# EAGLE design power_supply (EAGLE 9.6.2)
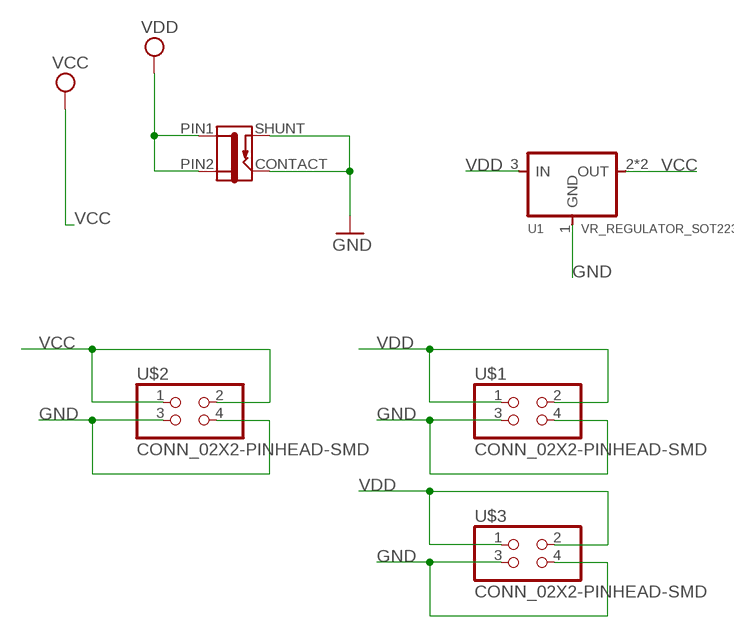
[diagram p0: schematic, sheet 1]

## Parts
J1  CONN_JACK-2.1MM  [PJ-002AH-SMT]
U1  VR_REGULATOR_SOT223  [SOT223]
U$1  CONN_02X2-PINHEAD-SMD  [2X02SMD]
U$2  CONN_02X2-PINHEAD-SMD  [2X02SMD]
U$3  CONN_02X2-PINHEAD-SMD  [2X02SMD]

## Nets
GND: J1.CONTACT J1.SHUNT U1.1(GND) U$1.3 U$1.4 U$2.3 U$2.4 U$3.3 U$3.4
VCC: U1.2(OUT) U1.4(OUT) U$2.1 U$2.2
VDD: J1.PIN1 J1.PIN2 U1.3(IN) U$1.1 U$1.2 U$3.1 U$3.2

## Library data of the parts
J1 = fab:CONN_JACK-2.1MM: SMD DC power jack PJ-002AH-SMT As found in the fablab inventory. Made by Zaerc.
U1 = fab:VR_REGULATOR_SOT223
U$1-U$3 = fab:CONN_02X2-PINHEAD-SMD

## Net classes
0 default: width 0.508 mm, clearance 0.508 mm

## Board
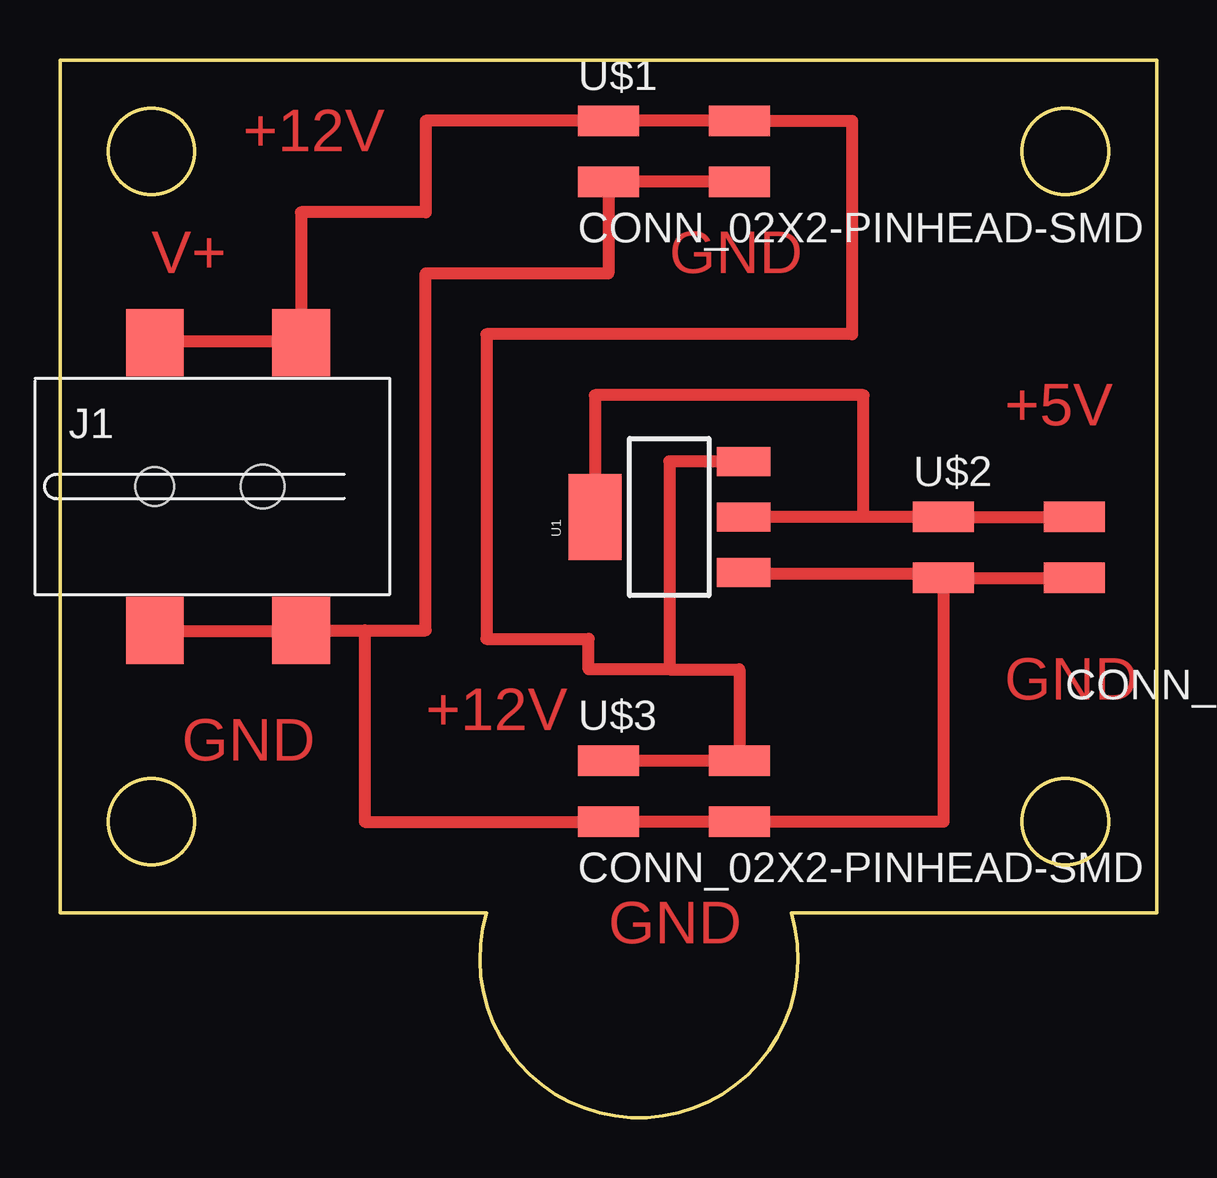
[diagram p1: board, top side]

Size 45.72 x 44.09 mm. Coordinates in mm from the lower left corner, seen from the top.
Outline: 45.72,8.53 45.72,44.09 0,44.09 0,8.53 17.78,8.53 arc213 30.48,8.53 45.72,8.53
Outline: circle at 3.81,12.34 radius 1.8
Outline: circle at 3.81,40.28 radius 1.8
Outline: circle at 41.91,40.28 radius 1.8
Outline: circle at 41.91,12.34 radius 1.8
Copper layers (1*16): Top 0.035mm / dielectric 1.5mm / Bottom 0.035mm
Design rules "default": minimum track width 6mil, minimum drill 0.35mm, track to track 6mil, track to pad 6mil, pad to pad 6mil, via to via 6mil, smd to smd 6mil, copper to edge 40mil, drill to drill 6mil, minimum pad ring 10mil, minimum via ring 8mil, stop-mask expansion 4mil, vias tented up to drill 0mil, thermal gap 10mil

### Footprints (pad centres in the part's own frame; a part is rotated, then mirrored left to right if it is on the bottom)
PJ-002AH-SMT = smd 2.4 x 2.8: CONTACT -2.4,-6; PIN1 3.7,6; PIN2 -2.4,6; SHUNT 3.7,-6 | hole 1.6: -2.4,0 | hole 1.8: 2.1,0
SOT223 = smd 1.219 x 2.235: 1 -2.311,-3.099; 2 0,-3.099; 3 2.311,-3.099 | smd 3.6 x 2.2: 4 0,3.099
2X02SMD = smd 2.54 x 1.27: 1 -2.54,1.27; 2 2.92,1.27; 3 -2.54,-1.27; 4 2.92,-1.27

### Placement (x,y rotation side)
J1  6.35,26.31 0 top
U1  25.4,25.04 90 top
U$1  25.4,40.28 0 top
U$2  39.37,23.77 0 top
U$3  25.4,13.61 0 top

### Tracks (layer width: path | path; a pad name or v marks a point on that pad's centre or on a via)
GND
  Top 0.508: U$2.3 36.67,22.66 28.57,22.66 U1.1 | U$2.3 U$2.4 | U$1.4 U$1.3 22.86,35.2 15.24,35.2 15.24,20.31 12.7,20.31 | J1.CONTACT 3.97,20.27 10,20.27 J1.SHUNT 12.7,20.31 | U$2.3 36.83,12.34 U$3.4 U$3.3 12.7,12.34 12.7,20.31
VCC
  Top 0.508: 33.5,25.04 U$2.1 U$2.2 | 33.5,25.04 U1.2 | 33.5,25.04 33.5,30.12 22.3,30.12 U1.4
VDD
  Top 0.508: J1.PIN2 3.97,32.34 10,32.34 J1.PIN1 10.05,37.74 15.24,37.74 15.24,41.55 U$1.1 U$1.2 33.02,41.55 33.02,32.66 17.78,32.66 17.78,19.96 22.03,19.96 22.03,18.69 25.4,18.69 | U1.3 25.4,27.35 25.4,18.69 | 25.4,18.69 28.32,18.69 U$3.2 U$3.1

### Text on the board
Top: +12V | V+ | GND | +5V | GND | +12V | GND | GND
